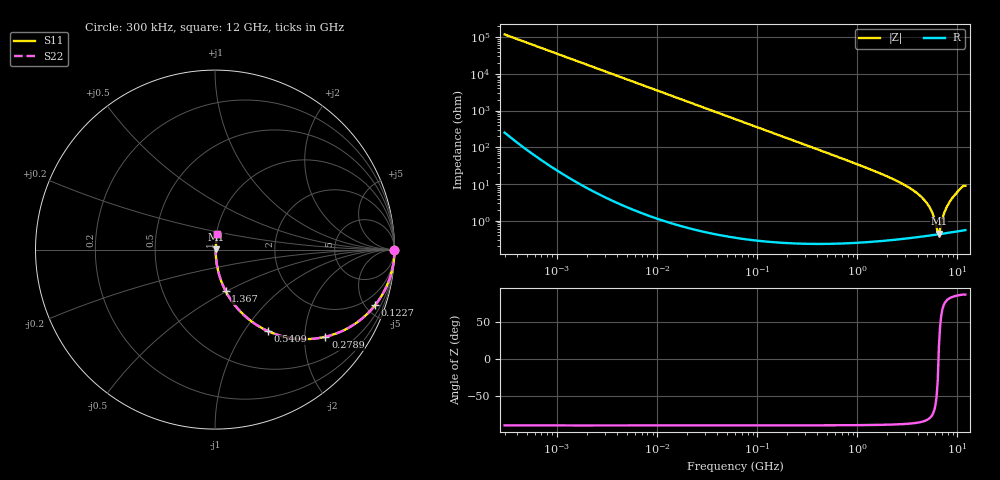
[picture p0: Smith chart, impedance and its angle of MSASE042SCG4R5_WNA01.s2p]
! MSASE042SCG4R5_WNA01  S-PARAMETER MODEL  ( General Type )
! Model Generated by TAIYO YUDEN Corporation (http://www.ty-top.com)
! Version 1.0
! TAIYO YUDEN Control No. 130801
! Copyright(c) 2013 TAIYO YUDEN CO.,LTD. All Rights Reserved.
! Product Description (link to TY-COMPAS)
! https://ds.yuden.co.jp/TYCOMPAS/or/detail?pn=MSASE042SCG4R5BWNA01&u=M
! Products Name : Multilayer Ceramic Capacitors
! Characteristics :
!  Capacitance : 4.5 pF , Rated Voltage : 16V , TCC : CG / C0G
!  Case Size : 0.4 x 0.2 / 0.016 x 0.008 [mm/inch] , Thickness : 0.2 / 0.008 [mm/inch]
!  (Conditions: Temperature = 25 degC , DC Bias Current/Voltage = 0A / 0V)
! External Node Assignments :
!  1  o---| |---o  2
! GND o---------o GND
! Frequency Range : 0.3MHz  -  12000MHz  [ 401 STEP ]
# MHz S RI R 50
! Freq[MHz].  S11 Real  S11 Imag  S21 Real  S21 Imag  S12 Real  S12 Imag  S22 Real  S22 Imag
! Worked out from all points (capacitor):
!   401 points, 300 kHz to 12 GHz, reference 50 ohm
!   read as one part in series: C = 4.5 pF near 316.3 kHz
!   lowest |Z| = 448 mohm at 6.525 GHz (marker M1)
!   series resonance near 6.467 GHz, so ESL is about 130 pH
!   S11 on the Smith chart (normalised r, x): 300 kHz: open; 122.7 MHz: 1.01, -5.76; 278.9 MHz: 1.00, -2.53; 540.9 MHz: 1.00, -1.30; 1.367 GHz: 1.01, -0.49; 12 GHz: 1.01, +0.18
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0.3  1 -0.000849  2.52e-06 0.000849  2.52e-06 0.000849  1 -0.000849
1.769972  1 -0.00501  2.74e-05 0.00501  2.74e-05 0.00501  1 -0.00501
10.44266  0.9991 -0.0295  0.000882 0.0295  0.000882 0.0295  0.9991 -0.0295
60  0.9719 -0.165  0.0281 0.165  0.0281 0.165  0.9719 -0.165
122.6847  0.8922 -0.3097  0.1078 0.3097  0.1078 0.3097  0.8922 -0.3097
278.9009  0.6152 -0.4856  0.3848 0.4856  0.3848 0.4856  0.6152 -0.4856
353.9943  0.4977 -0.4988  0.5023 0.4988  0.5023 0.4988  0.4977 -0.4988
540.8523  0.297 -0.4551  0.703 0.4551  0.703 0.4551  0.297 -0.4551
848.5281  0.1451 -0.3492  0.8549 0.3492  0.8549 0.3492  0.1451 -0.3492
1366.97  0.0598 -0.2317  0.9402 0.2317  0.9402 0.2317  0.0598 -0.2317
2088.533  0.0252 -0.1474  0.9748 0.1474  0.9748 0.1474  0.0252 -0.1474
3276.641  0.0097 -0.0793  0.9903 0.0793  0.9903 0.0793  0.0097 -0.0793
4502.883  0.00536 -0.0404  0.9946 0.0404  0.9946 0.0404  0.00536 -0.0404
5420.343  0.00438 -0.0196  0.9956 0.0196  0.9956 0.0196  0.00438 -0.0196
5715.274  0.00426 -0.0138  0.9957 0.0138  0.9957 0.0138  0.00426 -0.0138
6188.031  0.00423 -0.00517  0.9958 0.00517  0.9958 0.00517  0.00423 -0.00517
6524.734  0.00429 0.00122  0.9957 -0.00122  0.9957 -0.00122  0.00429 0.00122
6699.894  0.00435 0.00397  0.9957 -0.00397  0.9957 -0.00397  0.00435 0.00397
7448.838  0.0048 0.0167  0.9952 -0.0167  0.9952 -0.0167  0.0048 0.0167
8281.503  0.00568 0.0308  0.9943 -0.0308  0.9943 -0.0308  0.00568 0.0308
10511.28  0.0102 0.0702  0.9898 -0.0702  0.9898 -0.0702  0.0102 0.0702
12000  0.0133 0.0877  0.9867 -0.0877  0.9867 -0.0877  0.0133 0.0877
